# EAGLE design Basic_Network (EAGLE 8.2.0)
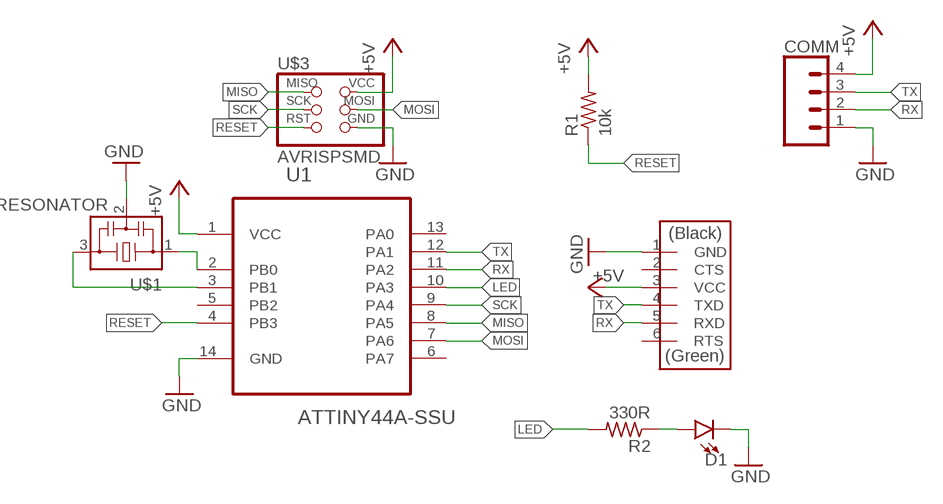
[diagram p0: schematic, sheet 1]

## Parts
COMM  CONN_04SMD  [1X04_SMD_RA_MALE]
D1  LED1206  [LED-1206]
FTDI  FTDI-SMD-HEADER  [1X06SMD]
R1  10k  R-US_R1206  [R1206]
R2  330R  R-US_R1206  [R1206]
U1  ATTINY44A-SSU  [SOIC127P600X175-14N]
U$1  RESONATOR  [EFOBM]
U$3  AVRISPSMD  [2X03SMD]

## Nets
+5V: COMM.4 FTDI.3(VCC) R1.2 U1.1(VCC) U$3.2(VCC)
GND: COMM.1 D1.C FTDI.1(GND) U1.14(GND) U$1.2 U$3.6(GND)
LED: R2.2 U1.10(PA3)
MISO: U1.8(PA5) U$3.1(MISO)
MOSI: U1.7(PA6) U$3.4(MOSI)
N$1: U1.2(PB0) U$1.1
N$2: U1.3(PB1) U$1.3
N$4: D1.A R2.1
RESET: R1.1 U1.4(PB3) U$3.5(RST)
RX: COMM.2 FTDI.5(RXD) U1.11(PA2)
SCK: U1.9(PA4) U$3.3(SCK)
TX: COMM.3 FTDI.4(TXD) U1.12(PA1)
Unconnected: FTDI.2(CTS) FTDI.6(RTS) U1.5(PB2) U1.6(PA7) U1.13(PA0)

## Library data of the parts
COMM = SparkFun-Connectors:CONN_04: Multi connection point. Often used as Generic Header-pin footprint for 0.1 inch spaced/style header connections On any of the 0.1 inch spaced packages, you can populate with these: Break Away Headers - Straight (PRT-00116) Break Away Male Headers - Right Angle (PRT-00553) Female Headers (PRT-00115)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; PROD_ID: CONN-09140; SF_ID: PRT-12638
D1 = SparkFun-LED:LED: LED (Generic)
FTDI = fab:FTDI-SMD-HEADER
R1 R2 = rcl:R-US_: RESISTOR, American symbol
U1 = Atmel_By_element14_Batch_1-00:ATTINY44A-SSU: 8-bit Microcontroller with In-System Programmable Flash; MPN: ATTINY44A-SSU; OC_FARNELL: 1699397; OC_NEWARK: 80P3683; PACKAGE: SOIC-14; SUPPLIER: Atmel
U$1 = fab:RESONATOR
U$3 = fab:AVRISP

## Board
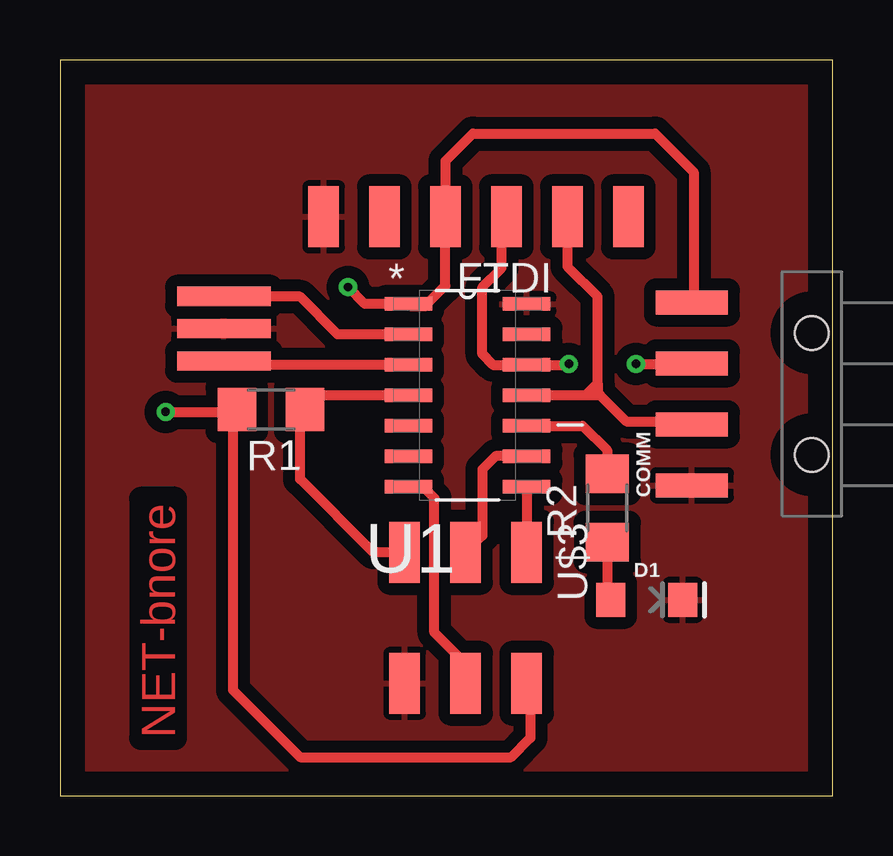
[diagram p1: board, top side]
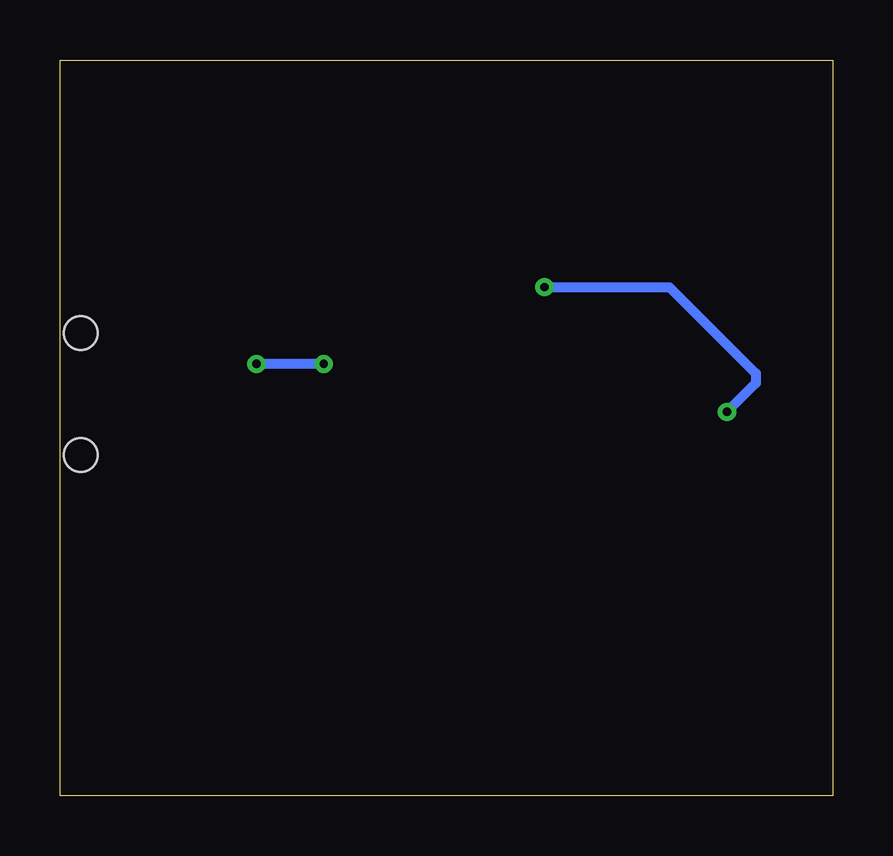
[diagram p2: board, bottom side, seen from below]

Size 32.19 x 30.67 mm. Coordinates in mm from the lower left corner, seen from the top.
Outline: 0,0 32.19,0 32.19,30.67 0,30.67 0,0
Copper layers (1*16): Top 0.035mm / dielectric 1.5mm / Bottom 0.035mm
Design rules "default *": minimum track width 6mil, minimum drill 0.35mm, track to track 0.4mm, track to pad 0.4mm, pad to pad 0.4mm, via to via 0.4mm, smd to smd 6mil, copper to edge 40mil, drill to drill 6mil, minimum pad ring 10mil, minimum via ring 8mil, stop-mask expansion 4mil, vias tented up to drill 0mil, thermal gap 10mil

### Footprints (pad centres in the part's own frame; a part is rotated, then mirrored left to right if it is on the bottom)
1X04_SMD_RA_MALE = smd 1 x 3: 1 -3.81,5; 2 -1.27,5; 3 1.27,5; 4 3.81,5 | hole 1.4: -2.54,0; 2.54,0
LED-1206 = smd 1.2 x 1.4: A -1.5,0; C 1.5,0
1X06SMD = smd 2.54 x 1.27: 1 0,6.35; 2 0,3.81; 3 0,1.27; 4 0,-1.27; 5 0,-3.81; 6 0,-6.35
R1206 = smd 1.6 x 1.803: 1 -1.422,0; 2 1.422,0
SOIC127P600X175-14N = smd 1.981 x 0.559: 1 -2.464,3.81; 2 -2.464,2.54; 3 -2.464,1.27; 4 -2.464,0; 5 -2.464,-1.27; 6 -2.464,-2.54; 7 -2.464,-3.81; 8 2.464,-3.81; 9 2.464,-2.54; 10 2.464,-1.27; 11 2.464,0; 12 2.464,1.27; 13 2.464,2.54; 14 2.464,3.81
EFOBM = smd 0.8 x 3.9: 1 -1.35,0; 2 0,0; 3 1.35,0
2X03SMD = smd 2.54 x 1.27: 1 -2.54,2.54; 2 2.92,2.54; 3 -2.54,0; 4 2.92,0; 5 -2.54,-2.54; 6 2.92,-2.54

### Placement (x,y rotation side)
COMM  31.33,16.75 90 top
D1  24.45,8.16 0 top
FTDI  17.33,24.13 90 top
R1  8.79,16.1 180 top
R2  22.8,11.99 90 top
U1  16.98,16.69 0 top
U$1  6.83,19.47 270 top
U$3  16.9,7.6 270 top

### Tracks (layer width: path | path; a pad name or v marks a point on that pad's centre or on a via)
+5V  (via drill 0.35)
  Top 0.406: 7.2,15.93 R1.2 | U$3.2 19.6,4.52 19.6,2.4 18.8,1.6 10,1.6 7.2,4.4 7.2,15.93 | COMM.4 26.4,20.63 26.4,26 24.8,27.6 17.2,27.6 16.06,26.46 FTDI.3 16.06,21.26 15.2,20.4 14.62,20.4 U1.1 12.7,20.5 v12,21.2 | v4.4,16 7.13,16 7.2,15.93
  Bottom 0.406: v12,21.2 6.8,21.2 3.2,17.6 3.2,17.2 v4.4,16
GND
  pour Top (isolate 0.5): 0,30.6 32.4,30.6 32.4,0 0,0
LED
  Top 0.406: U1.10 21.78,15.42 22.8,14.4 R2.2
MISO
  Top 0.406: U1.8 U$3.1
MOSI
  Top 0.406: U$3.4 16.9,5.5 15.6,6.8 15.6,12.4 15.2,12.8 14.6,12.8 U1.7
N$1
  Top 0.406: U1.2 11.57,19.23 10,20.8 6.85,20.8 U$1.1
N$2
  Top 0.406: U1.3 6.99,17.96 U$1.3
N$4
  Top 0.406: R2.1 22.8,8.31 D1.A
RESET
  Top 0.406: U1.4 10.8,16.69 R1.1 10,15.89 10,13.2 13.06,10.14 U$3.5
RX
  Top 0.406: 21.14,23.66 FTDI.5 21.14,22.06 22.4,20.8 22.4,17.2 | COMM.2 26.45,15.6 23.6,15.6 22.51,16.69 | 22.51,16.69 22,16.69 | 22,16.69 U1.11 | 22.4,17.2 22.4,16.8 22.51,16.69 | 22,16.69 22,16.8 22.4,17.2
SCK
  Top 0.406: U1.9 18.15,14.15 17.6,13.6 17.6,10.84 U$3.3
TX  (via drill 0.35)
  Top 0.406: U1.12 18.04,17.96 17.6,18.4 17.6,21.2 18.4,22 18.4,23.93 FTDI.4 | 19.5,18.02 U1.12 | COMM.3 26.27,17.96 26.23,18 v24,18 | U1.12 21.16,17.96 v21.2,18
  Bottom 0.406: v21.2,18 v24,18

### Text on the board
Top: NET-bnore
